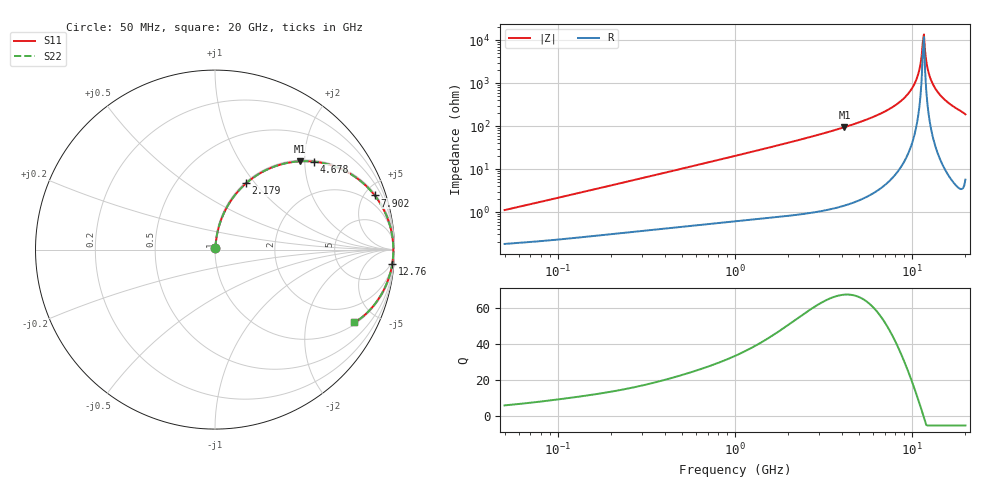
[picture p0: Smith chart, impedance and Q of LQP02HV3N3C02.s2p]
!Murata Part Number: LQP02HV3N3C02
!These Parameters are Measured in Series Mode Connection
!  o--[Z]--o
!Port1  Port2
!  o-------o
!Freq. Start=50[MHz] Stop=20[GHz], 401[Steps]
# Hz S RI R 50
!Freq.(Hz) S11(Real) S11(Imag) S21(Real) S21(Imag) S12(Real) S12(Imag) S22(Real) S22(Imag)
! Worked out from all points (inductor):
!   401 points, 50 MHz to 20 GHz, reference 50 ohm
!   read as one part in series: L = 3.45 nH near 51.52 MHz
!   highest Q = 67.1 at 4.149 GHz (marker M1), where L = 3.63 nH
!   self-resonance near 11.49 GHz
!   S11 on the Smith chart (normalised r, x): 50 MHz: 1.00, +0.02; 2.179 GHz: 1.02, +0.90; 4.678 GHz: 1.03, +2.22; 7.902 GHz: 1.14, +5.84; 12.76 GHz: 3, -24; 20 GHz: 1.11, -3.77
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5e7  0.00192 0.0109  0.9981 -0.0109  0.9981 -0.0109  0.00192 0.0109
1.364002e8  0.0034 0.0286  0.9966 -0.0286  0.9966 -0.0286  0.0034 0.0286
3.721004e8  0.00965 0.0752  0.9904 -0.0752  0.9904 -0.0752  0.00965 0.0752
1e9  0.0448 0.1924  0.9552 -0.1924  0.9552 -0.1924  0.0448 0.1924
2.179053e9  0.1735 0.3693  0.8265 -0.3693  0.8265 -0.3693  0.1735 0.3693
2.728004e9  0.2524 0.4261  0.7476 -0.4261  0.7476 -0.4261  0.2524 0.4261
4.149438e9  0.4731 0.4919  0.5269 -0.4919  0.5269 -0.4919  0.4731 0.4919
4.677679e9  0.5517 0.4899  0.4483 -0.4899  0.4483 -0.4899  0.5517 0.4899
7.442007e9  0.8578 0.3389  0.1422 -0.3389  0.1422 -0.3389  0.8578 0.3389
7.901521e9  0.8896 0.3019  0.1104 -0.3019  0.1104 -0.3019  0.8896 0.3019
9.178299e9  0.953 0.1949  0.047 -0.1949  0.047 -0.1949  0.953 0.1949
1.019291e10  0.9808 0.1107  0.0192 -0.1107  0.0192 -0.1107  0.9808 0.1107
1.082228e10  0.9898 0.0604  0.0102 -0.0604  0.0102 -0.0604  0.9898 0.0604
1.098561e10  0.9912 0.0477  0.0088 -0.0477  0.0088 -0.0477  0.9912 0.0477
1.131968e10  0.9931 0.0221  0.00691 -0.0221  0.00691 -0.0221  0.9931 0.0221
1.149051e10  0.9935 0.00929  0.00646 -0.00929  0.00646 -0.00929  0.9935 0.00929
1.183995e10  0.9934 -0.0164  0.00657 0.0164  0.00657 0.0164  0.9934 -0.0164
1.238412e10  0.9908 -0.0548  0.00922 0.0548  0.00922 0.0548  0.9908 -0.0548
1.276073e10  0.9874 -0.0802  0.0126 0.0802  0.0126 0.0802  0.9874 -0.0802
1.375312e10  0.9731 -0.1427  0.0269 0.1427  0.0269 0.1427  0.9731 -0.1427
1.504638e10  0.9456 -0.2142  0.0544 0.2142  0.0544 0.2142  0.9456 -0.2142
2e10  0.7736 -0.4037  0.2264 0.4037  0.2264 0.4037  0.7736 -0.4037
